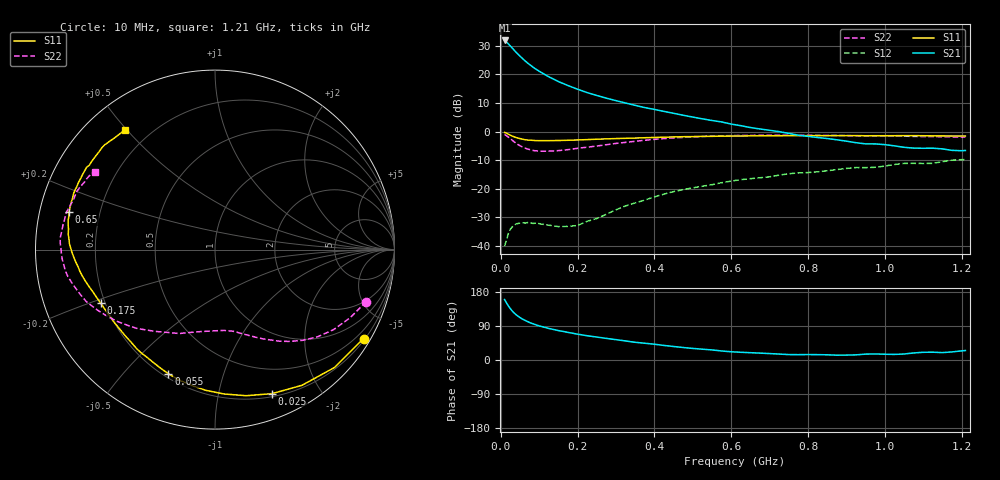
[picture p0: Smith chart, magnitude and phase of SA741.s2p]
!  POLYFET RF DEVICES
!  SA741
!  S PARAMETERS
!  VDS=50V, IDQ=200mA
# MHZ S MA R 50
! Freq=Mhz Mag[s11] Ang[s11] Mag[s21] Ang[s21] Mag[s12] Ang[s12] Mag[s22] Ang[s22]! Libra(R) for Windows Ver. 1.000.116.01  Cfg. (800 23205 1 3E8130A 32538 0 219F82
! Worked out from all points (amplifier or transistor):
!   64 points, 10 MHz to 1.21 GHz, reference 50 ohm
!   highest |S21| = 31.9 dB at 10 MHz (marker M1)
!   |S21| within 3 dB of that: start of sweep to 32.2 MHz
!   unconditionally stable (mu >= 1): 149.3 MHz to 294.5 MHz; 1.039 GHz to end of sweep
!   at 60 MHz: K = 0.32, MSG = 28.6 dB, |S12| = -32.0 dB
!   at 450 MHz: K = 0.68, MSG = 13.7 dB, |S12| = -21.1 dB
!   at 1.21 GHz: K = 1.11, MAG = -0.4 dB, |S12| = -9.8 dB
!   S11 on the Smith chart (normalised r, x): 10 MHz: 0.25, -3.60; 25 MHz: 0.23, -1.45; 55 MHz: 0.22, -0.67; 175 MHz: 0.18, -0.22; 650 MHz: 0.09, +0.13; 1.21 GHz: 0.11, +0.50
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10  0.9647 -30.9  39.36 159.4  0.00983 71.8  0.8909 -19.0
15  0.9348 -44.7  36.9 150.3  0.01265 67.2  0.8434 -26.8
20  0.8979 -57.4  34.15 142.5  0.01656 59.4  0.7968 -34.1
25  0.8631 -68.4  31.46 135.4  0.01951 52.3  0.7491 -40.5
30  0.8324 -78.0  28.93 129.1  0.0214 46.5  0.7028 -46.0
35  0.8058 -86.4  26.56 123.9  0.02286 42.0  0.6611 -50.7
40  0.7853 -93.9  24.39 119.4  0.02407 40.4  0.6241 -54.9
45  0.7671 -100.0  22.59 115.5  0.02461 36.4  0.5914 -58.4
55  0.7391 -110.5  19.46 108.9  0.02519 32.3  0.5434 -64.4
65  0.7169 -118.6  16.86 103.6  0.02493 29.2  0.5081 -69.4
75  0.7074 -125.5  14.93 98.9  0.02583 27.6  0.4832 -73.8
95  0.694 -135.3  11.96 91.6  0.02522 28.4  0.4576 -81.7
125  0.6929 -144.7  9.095 83.3  0.02289 33.3  0.4534 -91.9
175  0.7032 -154.8  6.386 72.9  0.02179 52.2  0.4821 -106.7
225  0.7225 -161.6  4.809 64.0  0.02681 77.2  0.5322 -119.9
325  0.7613 -170.6  3.163 50.3  0.04986 94.6  0.6462 -139.4
425  0.7964 -178.8  2.253 38.4  0.08017 96.5  0.7524 -155.1
625  0.8348 167.2  1.268 20.4  0.1434 87.7  0.8529 -176.4
650  0.8402 165.6  1.175 19.3  0.1495 86.1  0.8559 -178.6
825  0.8476 154.0  0.7864 14.1  0.1969 79.9  0.8549 169.0
1025  0.8451 139.8  0.5618 14.8  0.2647 74.5  0.8343 156.9
1210  0.8341 126.7  0.4662 24.9  0.3222 64.7  0.7986 147.0
